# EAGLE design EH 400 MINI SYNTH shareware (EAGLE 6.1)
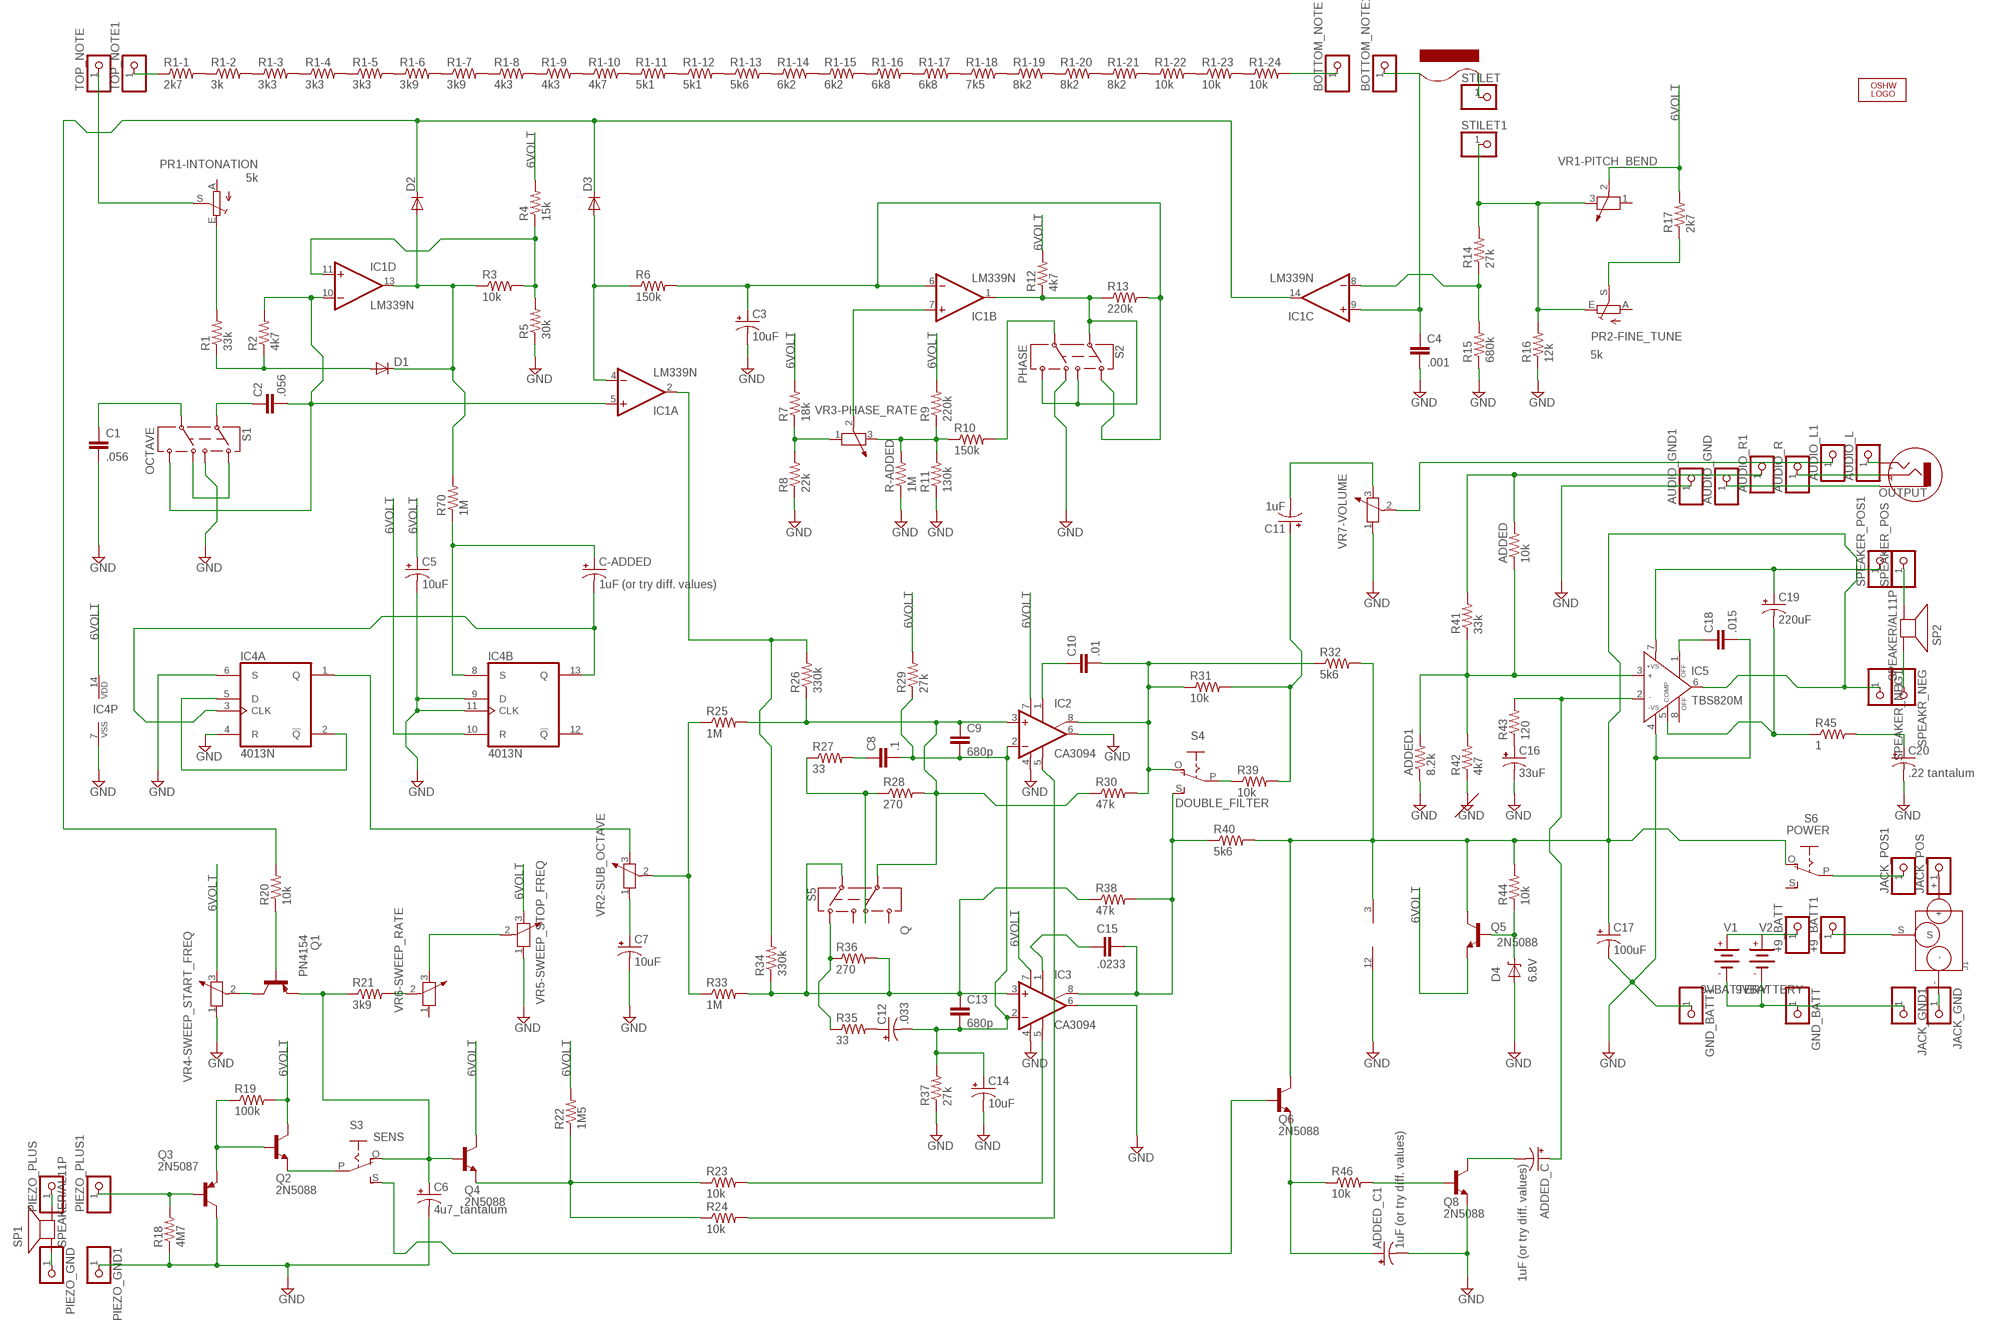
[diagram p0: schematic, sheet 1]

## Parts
+9_BATT  PINHD-1X1  [1X01]
+9_BATT1  PINHD-1X1  [1X01]
ADDED  10k  RESISTORPTH-1/4W  [AXIAL-0.4]
ADDED1  8.2k  RESISTORPTH-1/4W  [AXIAL-0.4]
ADDED_C  1uF (or try diff. values)  CAP_POLPTH2  [CPOL-RADIAL-10UF-25V]
ADDED_C1  1uF (or try diff. values)  CAP_POLPTH2  [CPOL-RADIAL-10UF-25V]
AUDIO_GND  PINHD-1X1  [1X01]
AUDIO_GND1  PINHD-1X1  [1X01]
AUDIO_L  PINHD-1X1  [1X01]
AUDIO_L1  PINHD-1X1  [1X01]
AUDIO_R  PINHD-1X1  [1X01]
AUDIO_R1  PINHD-1X1  [1X01]
BOTTOM_NOTE  PINHD-1X1  [1X01]
BOTTOM_NOTE1  PINHD-1X1  [1X01]
C1  .056  CAP_  [AXIAL-5MM]
C2  .056  CAP_  [AXIAL-5MM]
C3  10uF  CAP_POLPTH1  [CPOL-RADIAL-100UF-25V]
C4  .001  CAP_  [AXIAL-5MM]
C5  10uF  CAP_POLPTH2  [CPOL-RADIAL-10UF-25V]
C6  4u7_tantalum  CAP_POLPTH2  [CPOL-RADIAL-10UF-25V]
C7  10uF  CAP_POLPTH2  [CPOL-RADIAL-10UF-25V]
C8  .1  CAP_  [AXIAL-5MM]
C9  680p  CAP_  [AXIAL-5MM]
C10  .01  CAP_  [AXIAL-5MM]
C11  1uF  CAP_POLPTH1  [CPOL-RADIAL-100UF-25V]
C12  .033  CAP_POLPTH2  [CPOL-RADIAL-10UF-25V]
C13  680p  CAP_  [AXIAL-5MM]
C14  10uF  CAP_POLPTH2  [CPOL-RADIAL-10UF-25V]
C15  .0233  CAPPTH1  [CAP-PTH-5MM]
C16  33uF  CAP_POLPTH2  [CPOL-RADIAL-10UF-25V]
C17  100uF  CAP_POLPTH1  [CPOL-RADIAL-100UF-25V]
C18  .015  CAP_  [AXIAL-5MM]
C19  220uF  CAP_POLPTH1  [CPOL-RADIAL-100UF-25V]
C20  .22 tantalum  CAP_POLPTH1  [CPOL-RADIAL-100UF-25V]
C-ADDED  1uF (or try diff. values)  CAP_POLPTH2  [CPOL-RADIAL-10UF-25V]
D1  DIODE1N4148  [DIODE-1N4148]
D2  DIODE1N4148  [DIODE-1N4148]
D3  DIODE1N4148  [DIODE-1N4148]
D4  6.8V  DIODE-ZENERPTH  [DIODE-ZENER]
GND_BATT  PINHD-1X1  [1X01]
GND_BATT1  PINHD-1X1  [1X01]
IC1  LM339N  [DIL14]
IC2  CA3094  LM3080N  [DIL08]
IC3  CA3094  LM3080N  [DIL08]
IC4  4013N  [DIL14]
IC5  TBS820M  AD744N  [DIL08]
J1  JACK-3.5-3P  [PW-3P-3.5-14X9.5-DIP]
JACK_GND  PINHD-1X1  [1X01]
JACK_GND1  PINHD-1X1  [1X01]
JACK_POS  PINHD-1X1  [1X01]
JACK_POS1  PINHD-1X1  [1X01]
LOGO1  LOGO-OSHW-FILLX0200-NT  [OSHW_FILLX200_NOTEXT]
OUTPUT  AUDIO-JACK2.5MM  [STEREOJACK2.5MM_STEREOJACK2.5MM]
PIEZO_GND  PINHD-1X1  [1X01]
PIEZO_GND1  PINHD-1X1  [1X01]
PIEZO_PLUS  PINHD-1X1  [1X01]
PIEZO_PLUS1  PINHD-1X1  [1X01]
PR1-INTONATION  5k  TRIM_EU-S75P  [S75P]
PR2-FINE_TUNE  5k  TRIM_EU-S75P  [S75P]
Q1  PN4154  2N2907  [TO92-EBC-OVAL]
Q2  2N5088  2N2222  [TO92-EBC-OVAL]
Q3  2N5087  2N2907  [TO92-EBC-OVAL]
Q4  2N5088  2N2222  [TO92-EBC-OVAL]
Q5  2N5088  2N2222  [TO92-EBC-OVAL]
Q6  2N5088  2N2222  [TO92-EBC-OVAL]
Q8  2N5088  2N2222  [TO92-EBC-OVAL]
R1  33k  RESISTORPTH-1/4W  [AXIAL-0.4]
R1-1  2k7  RESISTORAXIAL-0.3  [AXIAL-0.3]
R1-2  3k  RESISTORAXIAL-0.3  [AXIAL-0.3]
R1-3  3k3  RESISTORAXIAL-0.3  [AXIAL-0.3]
R1-4  3k3  RESISTORAXIAL-0.3  [AXIAL-0.3]
R1-5  3k3  RESISTORAXIAL-0.3  [AXIAL-0.3]
R1-6  3k9  RESISTORAXIAL-0.3  [AXIAL-0.3]
R1-7  3k9  RESISTORAXIAL-0.3  [AXIAL-0.3]
R1-8  4k3  RESISTORAXIAL-0.3  [AXIAL-0.3]
R1-9  4k3  RESISTORAXIAL-0.3  [AXIAL-0.3]
R1-10  4k7  RESISTORAXIAL-0.3  [AXIAL-0.3]
R1-11  5k1  RESISTORAXIAL-0.3  [AXIAL-0.3]
R1-12  5k1  RESISTORAXIAL-0.3  [AXIAL-0.3]
R1-13  5k6  RESISTORAXIAL-0.3  [AXIAL-0.3]
R1-14  6k2  RESISTORAXIAL-0.3  [AXIAL-0.3]
R1-15  6k2  RESISTORAXIAL-0.3  [AXIAL-0.3]
R1-16  6k8  RESISTORAXIAL-0.3  [AXIAL-0.3]
R1-17  6k8  RESISTORAXIAL-0.3  [AXIAL-0.3]
R1-18  7k5  RESISTORAXIAL-0.3  [AXIAL-0.3]
R1-19  8k2  RESISTORAXIAL-0.3  [AXIAL-0.3]
R1-20  8k2  RESISTORAXIAL-0.3  [AXIAL-0.3]
R1-21  8k2  RESISTORAXIAL-0.3  [AXIAL-0.3]
R1-22  10k  RESISTORAXIAL-0.3  [AXIAL-0.3]
R1-23  10k  RESISTORAXIAL-0.3  [AXIAL-0.3]
R1-24  10k  RESISTORAXIAL-0.3  [AXIAL-0.3]
R2  4k7  RESISTORPTH-1/4W  [AXIAL-0.4]
R3  10k  RESISTORPTH-1/4W  [AXIAL-0.4]
R4  15k  RESISTORPTH-1/4W  [AXIAL-0.4]
R5  30k  RESISTORPTH-1/4W  [AXIAL-0.4]
R6  150k  RESISTORPTH-1/4W  [AXIAL-0.4]
R7  18k  RESISTORPTH-1/4W  [AXIAL-0.4]
R8  22k  RESISTORPTH-1/4W  [AXIAL-0.4]
R9  220k  RESISTORPTH-1/4W  [AXIAL-0.4]
R10  150k  RESISTORPTH-1/4W  [AXIAL-0.4]
R11  130k  RESISTORPTH-1/4W  [AXIAL-0.4]
R12  4k7  RESISTORPTH-1/4W  [AXIAL-0.4]
R13  220k  RESISTORPTH-1/4W  [AXIAL-0.4]
R14  27k  RESISTORPTH-1/4W  [AXIAL-0.4]
R15  680k  RESISTORPTH-1/4W  [AXIAL-0.4]
R16  12k  RESISTORPTH-1/4W  [AXIAL-0.4]
R17  2k7  RESISTORPTH-1/4W  [AXIAL-0.4]
R18  4M7  RESISTORPTH-1/4W  [AXIAL-0.4]
R19  100k  RESISTORPTH-1/4W  [AXIAL-0.4]
R20  10k  RESISTORPTH-1/4W  [AXIAL-0.4]
R21  3k9  RESISTORPTH-1/4W  [AXIAL-0.4]
R22  1M5  RESISTORPTH-1/4W  [AXIAL-0.4]
R23  10k  RESISTORPTH-1/4W  [AXIAL-0.4]
R24  10k  RESISTORPTH-1/4W  [AXIAL-0.4]
R25  1M  RESISTORPTH-1/4W  [AXIAL-0.4]
R26  330k  RESISTORPTH-1/4W  [AXIAL-0.4]
R27  33  RESISTORPTH-1/4W  [AXIAL-0.4]
R28  270  RESISTORPTH-1/4W  [AXIAL-0.4]
R29  27k  RESISTORPTH-1/4W  [AXIAL-0.4]
R30  47k  RESISTORPTH-1/4W  [AXIAL-0.4]
R31  10k  RESISTORPTH-1/4W  [AXIAL-0.4]
R32  5k6  RESISTORPTH-1/4W  [AXIAL-0.4]
R33  1M  RESISTORPTH-1/4W  [AXIAL-0.4]
R34  330k  RESISTORPTH-1/4W  [AXIAL-0.4]
R35  33  RESISTORPTH-1/4W  [AXIAL-0.4]
R36  270  RESISTORPTH-1/4W  [AXIAL-0.4]
R37  27k  RESISTORPTH-1/4W  [AXIAL-0.4]
R38  47k  RESISTORPTH-1/4W  [AXIAL-0.4]
R39  10k  RESISTORPTH-1/4W  [AXIAL-0.4]
R40  5k6  RESISTORPTH-1/4W  [AXIAL-0.4]
R41  33k  RESISTORPTH-1/4W  [AXIAL-0.4]
R42  4k7  RESISTORPTH-1/4W  [AXIAL-0.4]
R43  120  RESISTORPTH-1/4W  [AXIAL-0.4]
R44  10k  RESISTORPTH-1/4W  [AXIAL-0.4]
R45  1  RESISTORPTH-1/4W  [AXIAL-0.4]
R46  10k  RESISTORPTH-1/4W  [AXIAL-0.4]
R70  1M  RESISTORPTH-1/4W  [AXIAL-0.4]
R-ADDED  1M  RESISTORPTH-1/4W  [AXIAL-0.4]
S1  OCTAVE  SWITCH-DPDTOS  [OS]
S2  PHASE  SWITCH-DPDTOS  [OS]
S3  SENS  EG1218S  [EG1218]
S4  DOUBLE_FILTER  EG1218S  [EG1218]
S5  Q  SWITCH-DPDTOS  [OS]
S6  POWER  EG1218S  [EG1218]
SP1  SPEAKER/AL11P  [AL11P]
SP2  SPEAKER/AL11P  [AL11P]
SPEAKER_NEG1  PINHD-1X1  [1X01]
SPEAKER_POS  PINHD-1X1  [1X01]
SPEAKER_POS1  PINHD-1X1  [1X01]
SPEAKR_NEG  PINHD-1X1  [1X01]
STILET  PINHD-1X1  [1X01]
STILET1  PINHD-1X1  [1X01]
TOP_NOTE  PINHD-1X1  [1X01]
TOP_NOTE1  PINHD-1X1  [1X01]
V1  9VBATTERY  [AB9V]
V2  9VBATTERY  [AB9V]
VR1-PITCH_BEND  10k  R-POTENTIOMETER-3362U  [3362U]
VR2-SUB_OCTAVE  100k  R-POTENTIOMETER-3362U  [3362U]
VR3-PHASE_RATE  100k  R-POTENTIOMETER-3362U  [3362U]
VR4-SWEEP_START_FREQ  10k  R-POTENTIOMETER-3362U  [3362U]
VR5-SWEEP_STOP_FREQ  100k  R-POTENTIOMETER-3362U  [3362U]
VR6-SWEEP_RATE  100k  R-POTENTIOMETER-3362U  [3362U]
VR7-VOLUME  100k  R-POTENTIOMETER-3362U  [3362U]

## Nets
6VOLT: C5.1(+) IC2.7(V+) IC3.7(V+) IC4.10(B:R) IC4.14(P:VDD) Q2.C Q4.C Q5.E R4.P$2 R7.P$2 R9.P$2 R12.P$2 R17.P$2 R19.P$2 R22.P$2 R29.P$2 VR1-PITCH_BEND.2 VR4-SWEEP_START_FREQ.3 VR5-SWEEP_STOP_FREQ.3
GND: ADDED1.P$1 ADDED_C1.2(-) AUDIO_GND1.1 C1.P$2 C3.2(-) C4.P$2 C5.2(-) C6.2(-) C7.2(-) C14.2(-) C16.2(-) C17.2(-) C18.P$2 C20.2(-) D4.P$2(A) GND_BATT1.1 IC1.12(P:GND) IC2.4(V-) IC2.6(OUT) IC3.4(V-) IC3.6(OUT) IC4.4(A:R) IC4.6(A:S) IC4.7(P:VSS) IC4.9(B:D) IC4.11(B:CLK) IC5.4(-VS) PIEZO_GND1.1 Q3.C Q8.E R5.P$1 R8.P$1 R11.P$1 R15.P$1 R16.P$1 R18.P$1 R37.P$1 R42.P$1 R-ADDED.P$1 S1.3 S2.4 VR4-SWEEP_START_FREQ.1 VR5-SWEEP_STOP_FREQ.1 VR7-VOLUME.1
N$1: IC1.7(B:+IN) VR3-PHASE_RATE.2
N$2: C8.P$2 C9.P$2 C12.2(-) C13.P$2 C14.1(+) IC2.2(-IN) IC3.2(-IN) R29.P$1 R37.P$2
N$3: C7.1(+) VR2-SUB_OCTAVE.1
N$4: R7.P$1 R8.P$2 VR3-PHASE_RATE.1
N$5: C3.1(+) IC1.6(B:-IN) R6.P$2 R13.P$2 S2.1
N$6: D3.A IC1.4(A:-IN) R6.P$1
N$7: R10.P$2 S2.5
N$8: R9.P$1 R10.P$1 R11.P$2 R-ADDED.P$2 VR3-PHASE_RATE.3
N$9: IC1.2(A:OUT) R26.P$2 R34.P$2
N$10: D1.A R1.P$1 R2.P$1
N$11: C-ADDED.1(+) IC4.8(B:S) R70.P$1
N$12: AUDIO_L1.1 VR7-VOLUME.2
N$13: PR1-INTONATION.E R1.P$2
N$14: D1.C D2.A IC1.13(D:OUT) R3.P$1 R70.P$2
N$15: D2.C D3.C IC1.14(C:OUT) R20.P$2
N$16: IC1.11(D:+IN) R3.P$2 R4.P$1 R5.P$2
N$17: C-ADDED.2(-) IC4.3(A:CLK) IC4.13(B:Q)
N$18: R1-1.P$1 TOP_NOTE1.1
N$19: R1-1.P$2 R1-2.P$1
N$20: R1-2.P$2 R1-3.P$1
N$21: R1-3.P$2 R1-4.P$1
N$22: R1-4.P$2 R1-5.P$1
N$23: R1-5.P$2 R1-6.P$1
N$24: R1-6.P$2 R1-7.P$1
N$25: R1-7.P$2 R1-8.P$1
N$26: R1-8.P$2 R1-9.P$1
N$27: R1-9.P$2 R1-10.P$1
N$28: R1-10.P$2 R1-11.P$1
N$29: R1-11.P$2 R1-12.P$1
N$30: R1-12.P$2 R1-13.P$1
N$31: R1-15.P$2 R1-16.P$1
N$32: R1-16.P$2 R1-17.P$1
N$33: R1-17.P$2 R1-18.P$1
N$34: R1-18.P$2 R1-19.P$1
N$35: R1-19.P$2 R1-20.P$1
N$36: R1-13.P$2 R1-14.P$1
N$37: R1-14.P$2 R1-15.P$1
N$38: R1-20.P$2 R1-21.P$1
N$39: R1-21.P$2 R1-22.P$1
N$40: R25.P$1 R33.P$1 VR2-SUB_OCTAVE.2
N$41: R35.P$1 R36.P$1 S5.1
N$42: C9.P$1 IC2.3(+IN) R25.P$2 R26.P$1 R28.P$2 R30.P$1 S5.5
N$43: Q1.C VR4-SWEEP_START_FREQ.2
N$44: C13.P$1 IC3.3(+IN) R33.P$2 R34.P$1 R36.P$2 R38.P$1 S5.2
N$45: BOTTOM_NOTE1.1 C4.P$1 IC1.9(C:+IN)
N$46: PR2-FINE_TUNE.S R17.P$1
N$47: IC4.2(A:!Q) IC4.5(A:D)
N$48: IC4.1(A:Q) VR2-SUB_OCTAVE.3
N$49: IC1.1(B:OUT) R12.P$1 R13.P$1 S2.2 S2.3 S2.6
N$50: C1.P$1 S1.5
N$51: C2.P$1 S1.2
N$52: C2.P$2 IC1.5(A:+IN) IC1.10(D:-IN) R2.P$2 S1.6
N$53: S1.1 S1.4
N$54: Q1.B R20.P$1
N$55: C6.1(+) Q1.E Q4.B R21.P$1 S3.O
N$56: R21.P$2 VR6-SWEEP_RATE.2
N$57: VR5-SWEEP_STOP_FREQ.2 VR6-SWEEP_RATE.3
N$58: Q2.E S3.P
N$59: IC2.5(OPT) R24.P$2
N$60: Q2.B Q3.E R19.P$1
N$61: PIEZO_PLUS1.1 Q3.B R18.P$2
N$62: IC3.5(OPT) R23.P$2
N$63: Q4.E R22.P$1 R23.P$1 R24.P$1
N$64: IC1.8(C:-IN) R14.P$1 R15.P$2
N$65: PR2-FINE_TUNE.E R14.P$2 R16.P$2 STILET1.1 VR1-PITCH_BEND.3
N$66: C12.1(+) R35.P$2
N$67: C8.P$1 R27.P$2
N$68: R27.P$1 R28.P$1 S5.4
N$69: C10.P$1 IC2.1(ON1)
N$70: C15.1 IC3.1(ON1)
N$71: C15.2 IC3.8(ON2) R38.P$2 R40.P$1 S4.S
N$72: R39.P$1 S4.P
N$73: C10.P$2 IC2.8(ON2) R30.P$2 R31.P$1 R32.P$1 S4.O
N$74: C11.1(+) R31.P$2 R39.P$2
N$75: C17.1(+) IC1.3(P:V+) IC5.6(OUT) Q5.C Q6.C R32.P$2 R40.P$2 R44.P$2 S6.O SPEAKER_NEG1.1
N$76: C11.2(-) VR7-VOLUME.3
N$77: R1-22.P$2 R1-23.P$1
N$78: ADDED1.P$2 ADDED.P$1 IC5.3(IN+) R41.P$1 R42.P$2
N$79: ADDED.P$2 AUDIO_R1.1 R41.P$2
N$80: C18.P$1 IC5.1(OFF)
N$81: C19.1(+) IC5.7(+VS) SPEAKER_POS1.1
N$82: C19.2(-) IC5.5(COMP) R45.P$1
N$83: STILET.1
N$84: C20.1(+) R45.P$2
N$85: ADDED_C.1(+) IC5.2(IN-) R43.P$2
N$86: C16.1(+) R43.P$1
N$87: PIEZO_GND.1 SP1.+
N$88: PIEZO_PLUS.1 SP1.-
N$89: JACK_POS1.1 S6.P
N$90: +9_BATT.1 V1.+ V2.+
N$91: D4.P$1(C) Q5.B R44.P$1
N$92: SP2.- SPEAKER_POS.1
N$93: SP2.+ SPEAKR_NEG.1
N$94: J1.+ JACK_POS.1
N$95: +9_BATT1.1 J1.S
N$96: GND_BATT.1 JACK_GND1.1 V1.- V2.-
N$97: J1.- JACK_GND.1
N$98: AUDIO_L.1 OUTPUT.SHIELD(LEFT)
N$99: AUDIO_R.1 OUTPUT.TIP(RIGHT)
N$100: AUDIO_GND.1 OUTPUT.RING1(SLEEVE)
N$101: Q6.B S3.S
N$102: ADDED_C1.1(+) Q6.E R46.P$1
N$103: Q8.B R46.P$2
N$104: ADDED_C.2(-) Q8.C
N$105: R1-23.P$2 R1-24.P$1
N$106: BOTTOM_NOTE.1 R1-24.P$2
N$202: PR1-INTONATION.S TOP_NOTE.1
Unconnected: IC4.12(B:!Q) IC5.8(OFF) PR1-INTONATION.A PR2-FINE_TUNE.A S5.3 S5.6 S6.S VR1-PITCH_BEND.1 VR6-SWEEP_RATE.1

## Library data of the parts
+9_BATT +9_BATT1 AUDIO_GND AUDIO_GND1 AUDIO_L AUDIO_L1 AUDIO_R AUDIO_R1 BOTTOM_NOTE BOTTOM_NOTE1 GND_BATT GND_BATT1 JACK_GND JACK_GND1 JACK_POS JACK_POS1 PIEZO_GND PIEZO_GND1 PIEZO_PLUS PIEZO_PLUS1 SPEAKER_NEG1 SPEAKER_POS SPEAKER_POS1 SPEAKR_NEG STILET STILET1 TOP_NOTE TOP_NOTE1 = adafruit:PINHD-1X1: Pin header 1x1 for 0.1" spacing
ADDED ADDED1 R1 R1-1-R1-24 R2-R46 R70 R-ADDED = SparkFun:RESISTOR: Resistor
ADDED_C ADDED_C1 C3 C5-C7 C11 C12 C14 C16 C17 C19 C20 C-ADDED = SparkFun:CAP_POL: Capacitor Polarized
C1 C2 C4 C8-C10 C13 C15 C18 = SparkFun-MIRO:CAP: Capacitor
D1-D3 = SparkFun:DIODE: Diode
D4 = SparkFun:DIODE-ZENER: Zener Diode
IC1 = linear:LM339: Low Power Low Offset Voltage Quad Comparators with open collector; LM139/LM239/LM339/LM2901/LM3302
IC2 IC3 = linear:*3080: OP AMP
IC4 = 40xx:4013: Dual D FLIP FLOP, set/reset
IC5 = analog-devices:AD744: Precision, 500 ns Settling BiFET Op Amp Source: http://www.analog.com/static/imported-files/data_sheets/AD744.pdf; MF: ALTERA CORPORATION; MPN: AD744JNZ; OC_FARNELL: 1438362; OC_NEWARK: 59K4810
J1 = Connector:JACK-3.5-3P
LOGO1 = Logo:LOGO-OSHW-FILL
OUTPUT = SparkFun:AUDIO-JACK: 3.5mm Audio Jack Simple 3.5mm common PCB mount audio jack. SKU: PRT-08032
PR1-INTONATION PR2-FINE_TUNE = pot:TRIM_EU-: POTENTIOMETER
Q1 Q3 = adafruit:2N2907*: PNP Transistor Big Oval pads
Q2 Q4-Q6 Q8 = adafruit:2N2222: NPN TRANSISTOR Big oval pads
S1 S2 S5 = SparkFun-MIRO:SWITCH-DPDT: DPDT Version of the COM-00597
S3 S4 S6 = adafruit:EG1218: SLIDING SWITCH 0.1" spacing through hole, vertical SPDT slide switch http://www.ladyada.net/library/pcb/eaglelibrary.html
SP1 SP2 = adafruit:SPEAKER: SPEAKER
V1 V2 = gm-supply:9VBATTERY
VR1-PITCH_BEND VR2-SUB_OCTAVE VR3-PHASE_RATE VR4-SWEEP_START_FREQ VR5-SWEEP_STOP_FREQ VR6-SWEEP_RATE VR7-VOLUME = Discrete:R-POTENTIOMETER*: Potentiometer

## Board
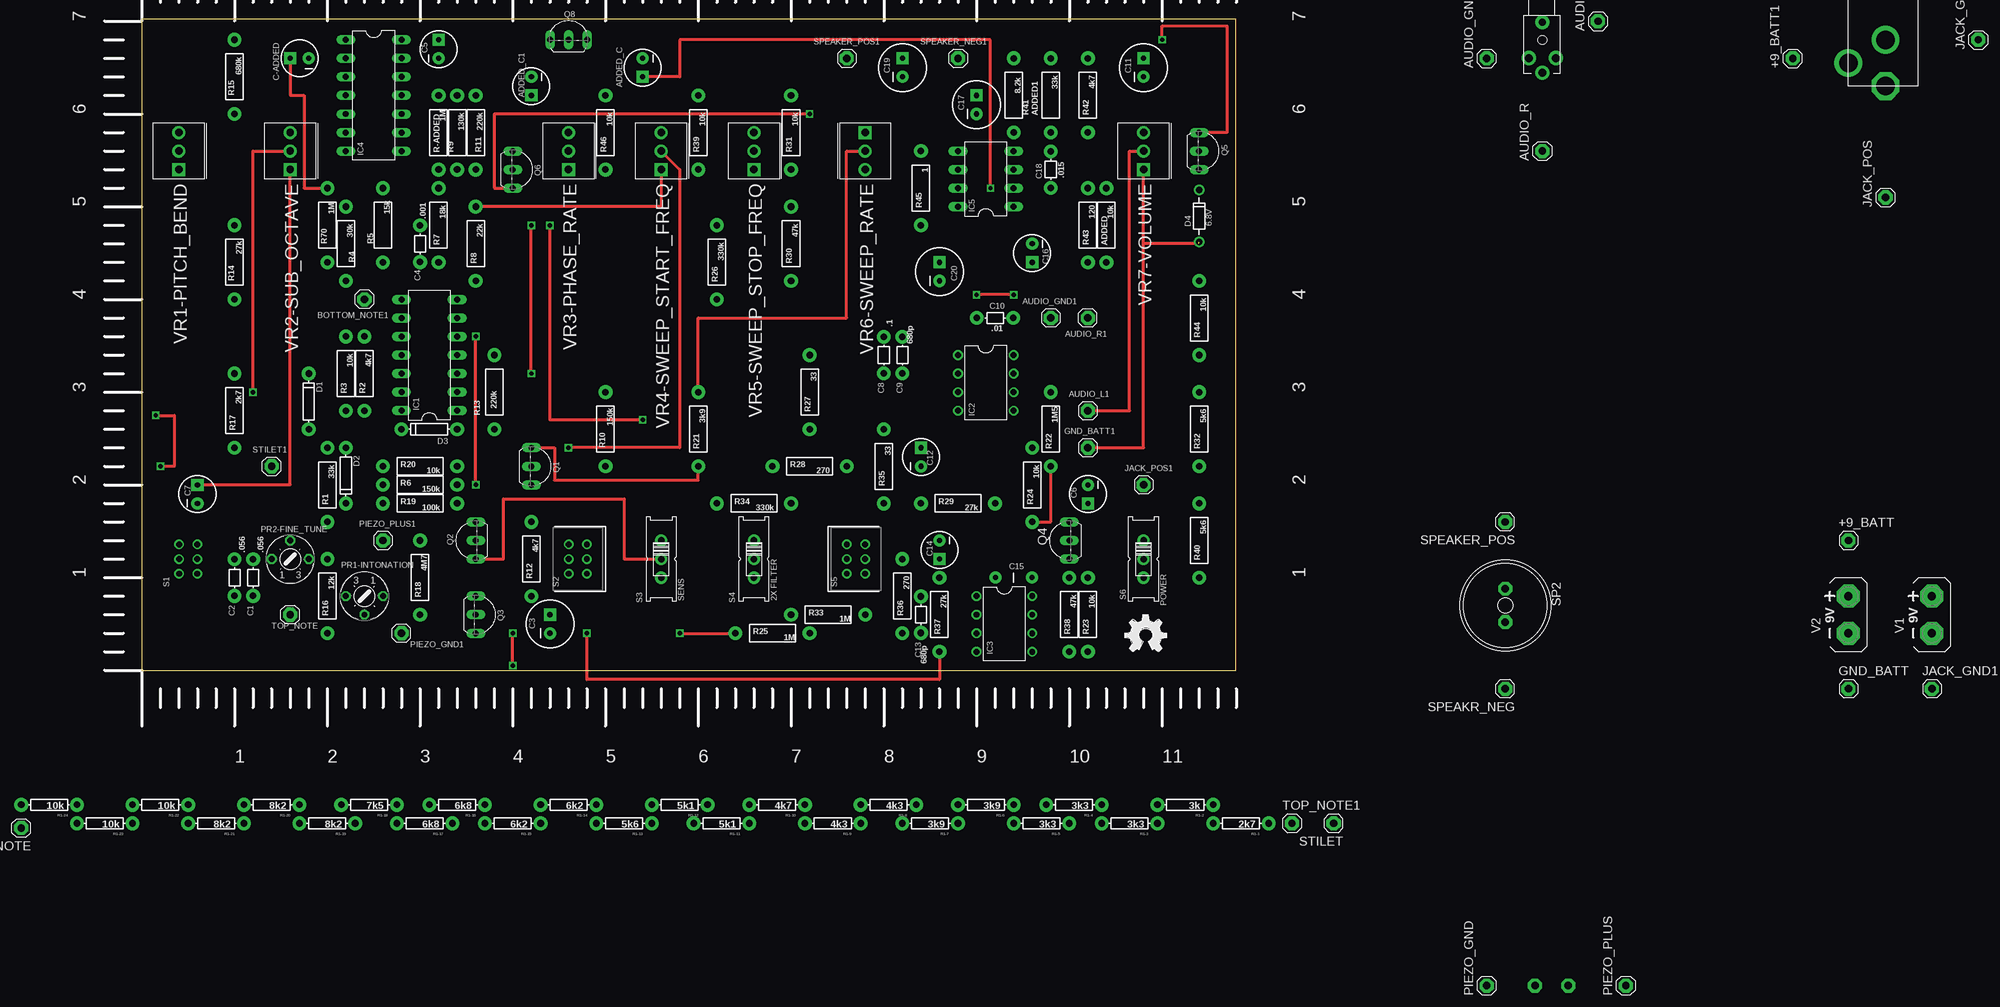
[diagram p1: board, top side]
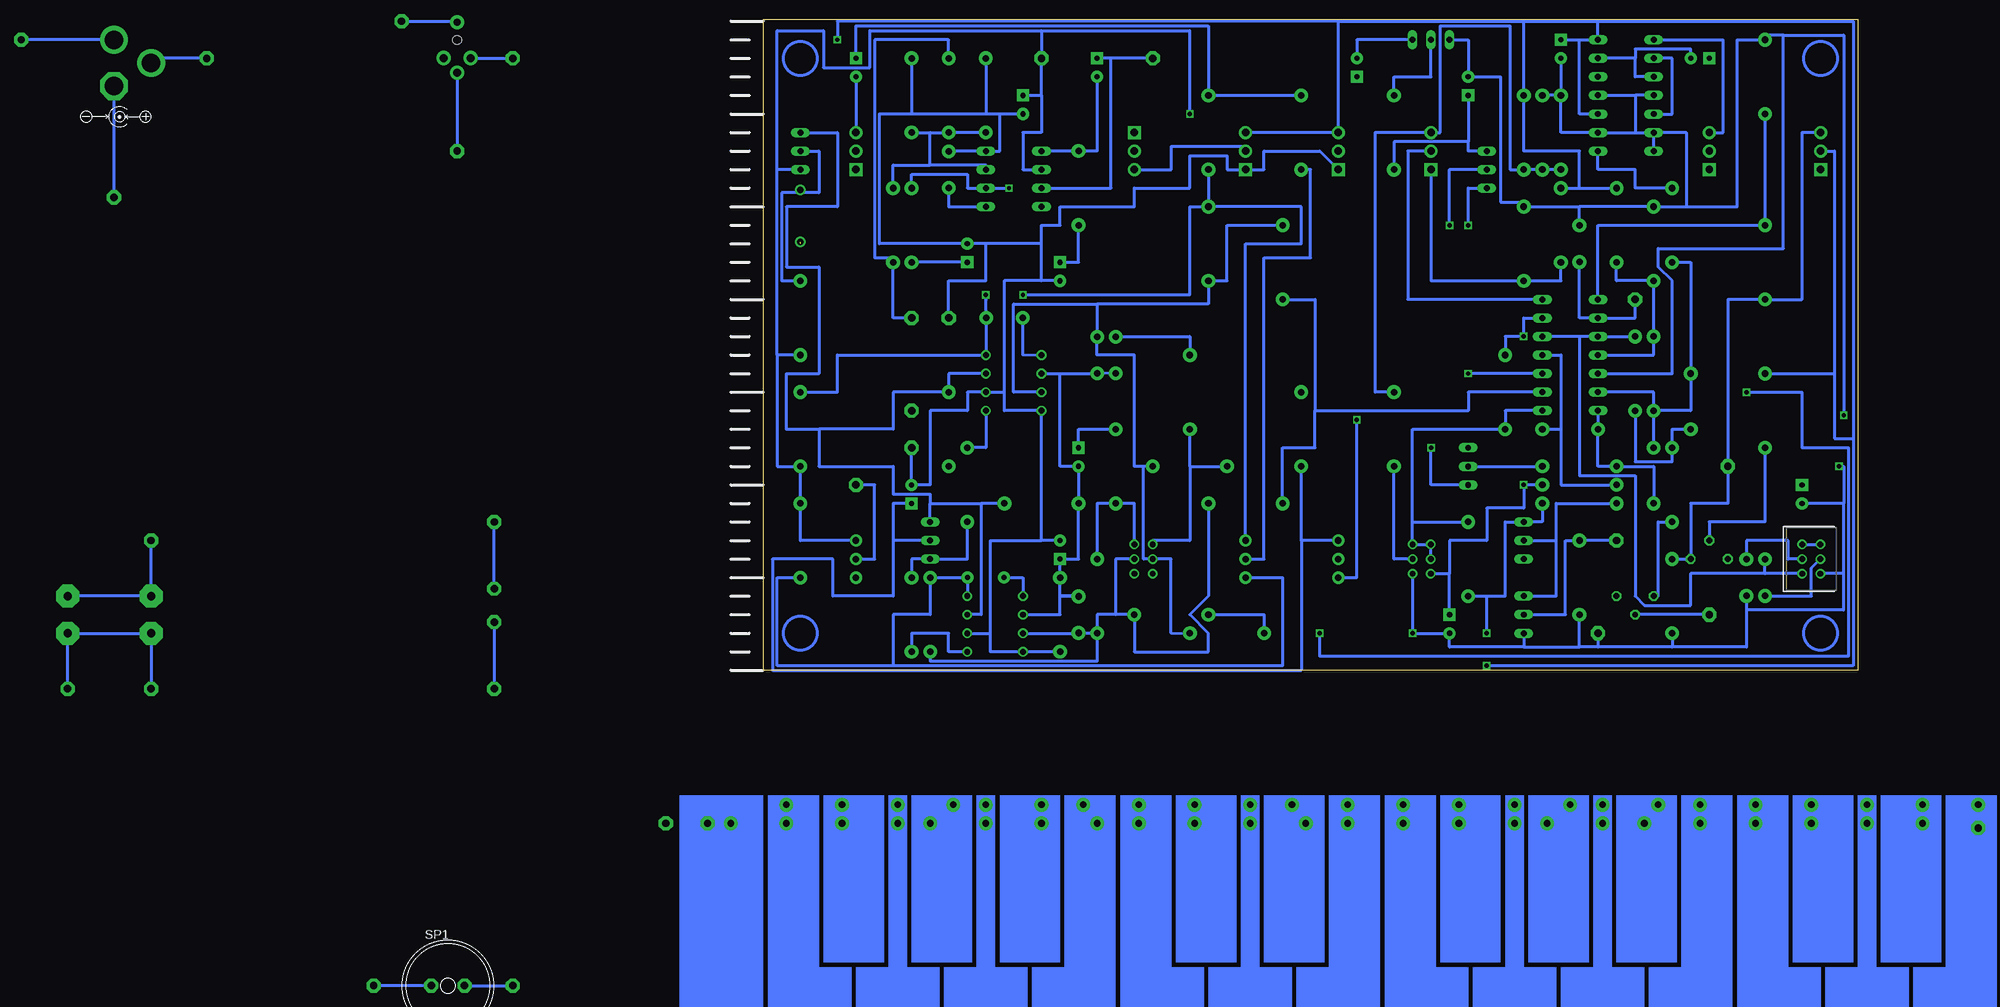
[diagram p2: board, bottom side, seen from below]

Size 149.84 x 89.2 mm. Coordinates in mm from the lower left corner, seen from the top.
Outline: 0,0 149.84,0 149.84,89.2 0,89.2 0,0
Copper layers (1*16): Top 0.035mm / dielectric 1.5mm / Bottom 0.035mm
Design rules: minimum track width 10mil, minimum drill 24mil, track to track 8mil, track to pad 8mil, pad to pad 8mil, via to via 8mil, smd to smd 8mil, copper to edge 40mil, drill to drill 8mil, minimum pad ring 10mil, minimum via ring 8mil, stop-mask expansion 4mil, vias tented up to drill 0mil, thermal gap 10mil

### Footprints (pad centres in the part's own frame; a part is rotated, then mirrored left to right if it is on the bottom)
1X01 = drill 1.016 pad 1.93 octagon: 1 0,0
AXIAL-0.4 = drill 0.9 pad 1.88: P$1 -5.08,0; P$2 5.08,0
CPOL-RADIAL-10UF-25V = drill 0.7 pad 1.651 square: 1 1.27,0 | drill 0.7 pad 1.651: 2 -1.27,0
AXIAL-5MM = drill 0.9 pad 1.88: P$1 -2.5,0; P$2 2.5,0
CPOL-RADIAL-100UF-25V = drill 0.7 pad 1.651 square: 1 1.27,0 | drill 0.7 pad 1.651: 2 -1.27,0
CAP-PTH-5MM = drill 0.7 pad 1.651: 1 -2.5,0; 2 2.5,0
DIODE-1N4148 = drill 0.9 pad 1.88: A -3.81,0; C 3.81,0
DIODE-ZENER = drill 0.9: P$1 -3.556,0; P$2 3.556,0
DIL14 = drill 0.813 long: 1 -7.62,-3.81; 2 -5.08,-3.81; 3 -2.54,-3.81; 4 0,-3.81; 5 2.54,-3.81; 6 5.08,-3.81; 7 7.62,-3.81; 8 7.62,3.81; 9 5.08,3.81; 10 2.54,3.81; 11 0,3.81; 12 -2.54,3.81; 13 -5.08,3.81; 14 -7.62,3.81
DIL08 = drill 0.813 pad 1.27: 1 -3.81,-3.81; 2 -1.27,-3.81; 3 1.27,-3.81; 4 3.81,-3.81; 5 3.81,3.81; 6 1.27,3.81; 7 -1.27,3.81; 8 -3.81,3.81
DIL08' = drill 0.813 long: 1 -3.81,-3.81; 2 -1.27,-3.81; 3 1.27,-3.81; 4 3.81,-3.81; 5 3.81,3.81; 6 1.27,3.81; 7 -1.27,3.81; 8 -3.81,3.81
PW-3P-3.5-14X9.5-DIP = drill 2.54 pad 3.81 octagon: + 0,0 | drill 2.54 pad 3.81: - -6.35,0; S -3.175,-5.08
STEREOJACK2.5MM_STEREOJACK2.5MM = drill 1.1 pad 1.93: RING1 2.5,-1.85; RING2 2.5,1.85; TIP 4.5,0 | drill 1 pad 1.93: SHIELD -2.4,0 | hole 1.2: 0,0
S75P = drill 0.813 octagon: A -2.54,0; E 2.54,0; S 0,2.54
TO92-EBC-OVAL = drill 0.813 long: B 0,-1.27; C 2.54,-1.27; E -2.54,-1.27
AXIAL-0.3 = drill 0.9 pad 1.88: P$1 -3.81,0; P$2 3.81,0
OS = drill 0.787 pad 1.27: 1 -2.007,1.245; 2 0,1.245; 3 2.007,1.245; 4 -2.007,-1.245; 5 0,-1.245; 6 2.007,-1.245
EG1218 = drill 0.9 pad 1.676: O -2.54,0; P 0,0; S 2.54,0
AL11P = drill 1.016 pad 1.905 octagon: + 2.286,0; - -2.286,0
AB9V = drill 1.118 pad 3.15 octagon: + 0,2.54; - 0,-2.54
3362U = drill 1.016 pad 1.778 square: 1 0,2.54 | drill 1.016 pad 1.778: 2 2.54,2.54; 3 5.08,2.54

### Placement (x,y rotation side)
+9_BATT  233.68,17.78 0 top  (outside the outline)
+9_BATT1  226.06,83.82 90 top  (outside the outline)
ADDED  132.08,60.96 270 top
ADDED1  119.38,78.74 270 top
ADDED_C  68.58,82.55 270 top
ADDED_C1  53.34,80.01 270 top
AUDIO_GND  184.15,83.82 90 top  (outside the outline)
AUDIO_GND1  124.46,48.26 0 top
AUDIO_L  199.39,88.9 90 top  (outside the outline)
AUDIO_L1  129.54,35.56 0 top
AUDIO_R  191.77,71.12 90 top  (outside the outline)
AUDIO_R1  129.54,48.26 180 top
BOTTOM_NOTE  -16.51,-21.59 180 top  (outside the outline)
BOTTOM_NOTE1  30.48,50.8 270 top
C1  15.24,12.7 270 top
C2  12.7,12.7 90 top
C3  55.88,6.35 90 top
C4  38.1,58.42 90 top
C5  40.64,85.09 90 top
C6  129.54,24.13 270 top
C7  7.62,24.13 90 top
C8  101.6,43.18 270 top
C9  104.14,43.18 270 top
C10  116.84,48.26 0 top
C11  137.16,82.55 90 top
C12  106.68,29.21 90 top
C13  106.68,7.62 90 top
C14  109.22,16.51 270 top
C15  119.38,12.7 0 top
C16  121.92,57.15 270 top
C17  114.3,77.47 90 top
C18  124.46,68.58 90 top
C19  104.14,82.55 90 top
C20  109.22,54.61 90 top
C-ADDED  21.59,83.82 180 top
D1  22.86,36.83 90 top
D2  27.94,26.67 270 top
D3  39.37,33.02 180 top
D4  144.78,62.23 270 top
GND_BATT  233.68,-2.54 0 top  (outside the outline)
GND_BATT1  129.54,30.48 0 top
IC1  39.37,43.18 90 top
IC2  115.57,39.37 270 top
IC3  118.11,6.35 270 top
IC4  31.75,78.74 270 top
IC5  TBS820M  [DIL08']  115.57,67.31 90 top
J1  238.76,80.01 270 top  (outside the outline)
JACK_GND  251.46,86.36 90 top  (outside the outline)
JACK_GND1  245.11,-2.54 0 top  (outside the outline)
JACK_POS  238.76,64.77 90 top  (outside the outline)
JACK_POS1  137.16,25.4 0 top
LOGO1  134.62,2.54 0 top
OUTPUT  191.77,86.36 270 top  (outside the outline)
PIEZO_GND  184.15,-43.18 90 top  (outside the outline)
PIEZO_GND1  35.56,5.08 180 top
PIEZO_PLUS  203.2,-43.18 90 top  (outside the outline)
PIEZO_PLUS1  33.02,17.78 0 top
PR1-INTONATION  30.48,10.16 180 top
PR2-FINE_TUNE  20.32,15.24 0 top
Q1  54.61,27.94 270 top
Q2  44.45,17.78 90 top
Q3  46.99,7.62 270 top
Q4  125.73,17.78 90 top
Q5  146.05,71.12 270 top
Q6  52.07,68.58 270 top
Q8  58.42,87.63 0 top
R1  25.4,25.4 270 top
R1-1  150.5,-20.96 180 top  (outside the outline)
R1-2  142.88,-18.41 180 top  (outside the outline)
R1-3  135.25,-20.96 180 top  (outside the outline)
R1-4  127.64,-18.41 180 top  (outside the outline)
R1-5  123.19,-20.96 180 top  (outside the outline)
R1-6  115.57,-18.41 180 top  (outside the outline)
R1-7  107.95,-20.96 180 top  (outside the outline)
R1-8  102.23,-18.41 180 top  (outside the outline)
R1-9  94.61,-20.96 180 top  (outside the outline)
R1-10  87,-18.41 180 top  (outside the outline)
R1-11  79.38,-20.96 180 top  (outside the outline)
R1-12  73.66,-18.41 180 top  (outside the outline)
R1-13  66.04,-20.96 180 top  (outside the outline)
R1-14  58.42,-18.41 180 top  (outside the outline)
R1-15  50.8,-20.96 180 top  (outside the outline)
R1-16  43.18,-18.41 180 top  (outside the outline)
R1-17  38.73,-20.96 180 top  (outside the outline)
R1-18  31.11,-18.41 180 top  (outside the outline)
R1-19  25.4,-20.96 180 top  (outside the outline)
R1-20  17.78,-18.41 180 top  (outside the outline)
R1-21  10.16,-20.96 180 top  (outside the outline)
R1-22  2.54,-18.41 180 top  (outside the outline)
R1-23  -5.08,-20.96 180 top  (outside the outline)
R1-24  -12.7,-18.41 180 top  (outside the outline)
R2  30.48,40.64 90 top
R3  27.94,40.64 90 top
R4  33.02,60.96 90 top
R5  27.94,58.42 270 top
R6  38.1,25.4 0 top
R7  40.64,60.96 90 top
R8  45.72,58.42 270 top
R9  45.72,73.66 90 top
R10  63.5,33.02 270 top
R11  43.18,73.66 270 top
R12  53.34,15.24 270 top
R13  48.26,38.1 90 top
R14  12.7,55.88 270 top
R15  12.7,81.28 270 top
R16  25.4,10.16 90 top
R17  12.7,35.56 90 top
R18  38.1,12.7 90 top
R19  38.1,22.86 0 top
R20  38.1,27.94 180 top
R21  76.2,33.02 90 top
R22  124.46,33.02 90 top
R23  129.54,7.62 270 top
R24  121.92,25.4 90 top
R25  86.36,5.08 0 top
R26  78.74,55.88 270 top
R27  91.44,38.1 90 top
R28  91.44,27.94 0 top
R29  111.76,22.86 0 top
R30  88.9,58.42 90 top
R31  88.9,73.66 90 top
R32  144.78,33.02 270 top
R33  93.98,7.62 0 top
R34  83.82,22.86 180 top
R35  101.6,27.94 90 top
R36  104.14,10.16 270 top
R37  109.22,7.62 90 top
R38  127,7.62 90 top
R39  76.2,73.66 90 top
R40  144.78,17.78 90 top
R41  124.46,78.74 90 top
R42  129.54,78.74 270 top
R43  129.54,60.96 90 top
R44  144.78,48.26 270 top
R45  106.68,66.04 270 top
R46  63.5,73.66 90 top
R70  25.4,60.96 270 top
R-ADDED  40.64,73.66 270 top
S1  6.35,15.24 270 bottom
S2  59.69,15.24 90 top
S3  71.12,15.24 270 top
S4  83.82,15.24 270 top
S5  97.79,15.24 270 top
S6  137.16,15.24 270 top
SP1  193.04,-43.18 0 bottom  (outside the outline)
SP2  186.69,8.89 270 top  (outside the outline)
SPEAKER_NEG1  111.76,83.82 0 top
SPEAKER_POS  186.69,20.32 180 top  (outside the outline)
SPEAKER_POS1  96.52,83.82 0 top
SPEAKR_NEG  186.69,-2.54 180 top  (outside the outline)
STILET  not placed on the board
STILET1  17.78,27.94 90 top
TOP_NOTE  20.32,7.62 180 top
TOP_NOTE1  157.48,-20.96 0 top  (outside the outline)
V1  245.11,7.62 0 top  (outside the outline)
V2  233.68,7.62 0 top  (outside the outline)
VR1-PITCH_BEND  7.62,68.58 90 top
VR2-SUB_OCTAVE  22.86,68.58 90 top
VR3-PHASE_RATE  60.96,68.58 90 top
VR4-SWEEP_START_FREQ  73.66,68.58 90 top
VR5-SWEEP_STOP_FREQ  86.36,68.58 90 top
VR6-SWEEP_RATE  96.52,73.66 270 top
VR7-VOLUME  139.7,68.58 90 top

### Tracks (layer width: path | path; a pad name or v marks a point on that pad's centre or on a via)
6VOLT  (via drill 0.6)
  Top 0.406: v139.7,86.36 139.7,88.27 148.59,88.27 148.59,73.66 Q5.E | v50.8,0.64 v50.8,5.08
  Bottom 0.406: Q5.E 139.7,73.66 139.7,63.5 146.69,63.5 146.69,55.25 142.24,55.25 142.24,40.64 146.69,40.64 146.69,33.02 142.24,33.02 | 127,22.86 127,24.13 132.08,24.13 132.08,27.94 142.24,27.94 142.24,33.02 | Q4.C 127,22.86 | 127,22.86 120.02,22.86 | R29.P$2 120.02,22.86 | 120.02,22.86 120.02,7.62 IC3.7 | IC2.7 124.46,40.64 R22.P$2 132.08,38.1 132.08,33.02 142.24,33.02 | 71.12,88.9 VR4-SWEEP_START_FREQ.3 VR5-SWEEP_STOP_FREQ.3 | 71.12,88.9 139.7,88.9 v139.7,86.36 | C5.1 38.1,86.36 | R19.P$2 43.18,20.32 Q2.C 48.26,20.32 48.26,10.16 50.8,10.16 | 45.72,88.9 35.56,88.9 | 35.56,88.9 0.64,88.9 0.64,31.75 | 38.1,66.04 38.1,71.12 45.72,71.12 R9.P$2 45.72,88.9 | VR1-PITCH_BEND.2 3.17,71.12 3.17,40.64 | 3.17,40.64 3.17,31.75 0.64,31.75 | 0.64,31.75 0.64,0.64 v50.8,0.64 | 71.12,88.9 45.72,88.9 | IC4.10 38.1,76.2 38.1,86.36 | 38.1,86.36 IC4.14 35.56,88.9 | R12.P$2 50.8,10.16 | v50.8,5.08 50.8,10.16 | R7.P$2 38.1,66.04 | 38.1,66.04 R4.P$2 | R17.P$2 3.17,40.64
GND  (via drill 0.6)  (1 unrouted)
  Top 0.406: v1.91,34.93 4.45,34.93 4.45,27.94 v2.54,27.94 | R37.P$1 109.22,-1.27 60.96,-1.27 v60.96,5.08 | GND_BATT1.1 137.16,30.48 137.16,58.42 | 137.16,58.42 VR7-VOLUME.1 | VR4-SWEEP_START_FREQ.1 71.12,63.5 R8.P$1 | 144.78,58.42 137.16,58.42
  Bottom 0.406: IC4.7 IC4.6 | IC4.4 30.48,78.74 | 30.48,78.74 30.48,73.66 | 30.48,73.66 IC4.6 | R-ADDED.P$1 40.64,73.66 IC4.9 30.48,73.66 | IC4.11 30.48,78.74 | IC4.6 23.5,73.66 23.5,63.5 | 10.16,86.99 1.91,86.99 v1.91,34.93 | v2.54,27.94 1.91,27.94 1.91,22.86 | IC1.12 25.4,40.64 25.4,53.34 27.3,55.25 27.3,57.79 10.16,57.79 10.16,86.99 | 10.16,86.99 12.7,86.99 R15.P$1 16.51,86.36 16.51,63.5 23.5,63.5 | 38.1,63.5 R8.P$1 45.72,64.13 48.9,64.13 48.9,81.28 ADDED_C1.2 53.34,86.36 Q8.E | 23.5,63.5 R5.P$1 38.1,63.5 | C5.2 R-ADDED.P$1 | R-ADDED.P$1 R11.P$1 | C4.P$2 38.1,63.5 | 1.91,22.86 C7.2 8.26,22.86 | 1.91,13.33 1.91,22.86 | 15.24,8.25 1.91,8.25 1.91,13.33 | C1.P$2 15.24,8.25 | 15.24,8.25 15.24,3.17 25.4,3.17 | R16.P$1 25.4,3.17 | 25.4,3.17 35.56,3.17 | PIEZO_GND1.1 35.56,3.17 | 45.72,3.17 38.1,3.17 | 35.56,3.17 38.1,3.17 | 38.1,3.17 R18.P$1 | Q3.C 45.72,3.17 | 45.72,3.17 55.88,3.17 C3.2 v60.96,5.08 | 60.96,4.95 v60.96,5.08 | v60.96,5.08 60.94,5.1 S2.4 | 117.47,76.2 117.47,71.12 IC5.4 124.46,71.12 C18.P$2 | C17.2 117.47,76.2 | 117.47,76.2 119.38,76.2 | 119.38,76.2 129.54,76.2 | R42.P$1 129.54,76.2 | 129.54,76.2 133.99,76.2 133.99,58.42 C16.2 119.38,58.42 | 111.76,53.34 116.84,53.34 116.84,38.1 | 111.76,53.34 111.76,58.42 | 111.76,58.42 119.38,58.42 | C20.2 111.76,53.34 | 111.76,58.42 111.76,60.96 109.22,60.96 109.22,63.5 99.06,63.5 99.06,66.04 91.44,66.04 91.44,70.48 86.36,70.48 86.36,68.58 VR5-SWEEP_STOP_FREQ.1 81.28,68.58 81.28,71.12 73.66,71.12 VR4-SWEEP_START_FREQ.1 | IC3.6 118.75,5.08 | 118.75,5.08 118.75,2.54 IC3.4 R37.P$1 | 118.75,5.08 118.75,17.78 111.76,17.78 | C14.2 111.76,17.78 | 111.76,17.78 IC2.4 116.84,35.56 116.84,38.1
  Bottom 0.406: 116.84,38.1 IC2.6 121.92,38.1 121.92,35.56 127,35.56 127,25.4 C6.2 GND_BATT1.1 | ADDED1.P$1 119.38,76.2 | AUDIO_GND1.1 124.46,53.34 119.38,53.34 119.38,58.42 | S1.3 5.11,13.33 1.91,13.33
N$1
  Bottom 0.406: IC1.7 61.59,50.8 61.59,71.12 VR3-PHASE_RATE.2
N$2
  Bottom 0.406: 109.22,10.16 C13.P$2 106.68,10.16 109.22,10.16 | IC3.2 109.22,7.62 109.22,10.16 | 109.22,10.16 R37.P$2 C14.1 106.68,15.24 R29.P$1 C12.2 109.22,27.94 109.22,40.64 | 109.22,40.64 C9.P$2 | C8.P$2 101.6,40.64 C9.P$2 | IC2.2 109.22,40.64 | 109.22,40.64 104.14,40.64 C9.P$2
N$3
  Top 0.406: VR2-SUB_OCTAVE.1 20.32,25.4 C7.1
N$4
  Bottom 0.406: VR3-PHASE_RATE.1 58.42,53.34 R8.P$2 40.64,53.34 R7.P$1
N$5  (via drill 0.6)
  Top 0.406: v45.72,25.4 v45.72,45.72
  Bottom 0.406: IC1.6 45.72,48.26 v45.72,45.72 48.26,45.72 R13.P$2 | R6.P$2 v45.72,25.4 45.72,22.22 50.8,22.22 50.8,17.78 55.88,17.78 55.88,13.23 | S2.1 55.88,13.23 | C3.1 55.88,13.23
N$6
  Bottom 0.406: IC1.4 40.64,43.18 40.64,33.02 | D3.A 40.64,33.02 | 40.64,33.02 40.64,25.4 R6.P$1
N$7
  Bottom 0.406: S2.5 63.5,15.24 R10.P$2
N$8
  Bottom 0.406: R-ADDED.P$2 R11.P$2 R9.P$1 47.62,68.58 47.62,88.27 57.15,88.27 57.15,73.66 VR3-PHASE_RATE.3 66.04,73.66 66.04,38.1 R10.P$1
N$9
  Bottom 0.406: IC1.2 53.34,38.1 53.34,35.56 74.3,35.56 | R26.P$2 74.3,50.8 74.3,35.56 | R34.P$2 78.74,30.48 74.3,30.48 74.3,35.56
N$10
  Bottom 0.406: D1.A 25.4,33.02 R1.P$1 25.4,28.57 30.48,28.57 R2.P$1
N$11
  Top 0.406: C-ADDED.1 20.32,78.74 22.23,78.74 22.23,66.04 R70.P$1
  Bottom 0.406: R70.P$1 30.48,66.04 30.48,68.58 35.56,68.58 IC4.8
N$12
  Top 0.406: AUDIO_L1.1 135.25,35.56 135.25,71.12 VR7-VOLUME.2
N$13
  Bottom 0.406: PR1-INTONATION.E 27.3,10.16 27.3,20.32 R1.P$2
N$14
  Bottom 0.406: R3.P$1 27.94,38.1 IC1.13 | R70.P$2 22.86,55.88 D1.C 22.86,35.56 R3.P$1 | D2.A R3.P$1
N$15
  Bottom 0.406: D2.C 27.94,27.94 R20.P$2 35.56,27.94 D3.C IC1.14
N$16
  Bottom 0.406: IC1.11 27.94,43.18 R3.P$2 R5.P$2 33.02,53.34 R4.P$1
N$17
  Bottom 0.406: IC4.3 30.48,81.28 30.48,83.82 | 30.48,83.82 IC4.13 | C-ADDED.2 22.86,85.09 30.48,85.09 30.48,83.82
N$18
  Bottom 0.406: TOP_NOTE1.1 R1-1.P$1
N$19
  Bottom 0.406: R1-1.P$2 R1-2.P$1
N$20
  Bottom 0.406: R1-2.P$2 R1-3.P$1
N$21
  Bottom 0.406: R1-3.P$2 R1-4.P$1
N$22
  Bottom 0.406: R1-4.P$2 127,-18.41 R1-5.P$1
N$23
  Bottom 0.406: R1-6.P$1 R1-5.P$2
N$24
  Bottom 0.406: R1-7.P$1 R1-6.P$2
N$25
  Bottom 0.406: R1-8.P$1 104.14,-18.41 R1-7.P$2
N$26
  Bottom 0.406: R1-8.P$2 R1-9.P$1
N$27
  Bottom 0.406: R1-9.P$2 R1-10.P$1
N$28
  Bottom 0.406: R1-10.P$2 R1-11.P$1
N$29
  Bottom 0.406: R1-12.P$1 75.56,-18.41 R1-11.P$2
N$30
  Bottom 0.406: R1-12.P$2 R1-13.P$1
N$31
  Bottom 0.406: R1-16.P$1 R1-15.P$2
N$32
  Bottom 0.406: R1-16.P$2 42.55,-18.41 R1-17.P$1
N$33
  Bottom 0.406: R1-17.P$2 R1-18.P$1
N$34
  Bottom 0.406: R1-18.P$2 29.21,-18.41 R1-19.P$1
N$35
  Bottom 0.406: R1-20.P$1 R1-19.P$2
N$36
  Bottom 0.406: R1-14.P$1 R1-13.P$2
N$37
  Bottom 0.406: R1-14.P$2 R1-15.P$1
N$38
  Bottom 0.406: R1-20.P$2 R1-21.P$1
N$39
  Bottom 0.406: R1-22.P$1 R1-21.P$2
N$40  (via drill 0.6)
  Top 0.406: v73.66,5.08 R25.P$1 | v15.24,38.1 15.24,71.12 VR2-SUB_OCTAVE.2
  Bottom 0.406: v15.24,38.1 7.62,38.1 7.62,30.48 1.27,30.48 1.27,1.91 73.66,1.91 v73.66,5.08 | R33.P$1 81.28,7.62 R25.P$1
N$41
  Bottom 0.406: R36.P$1 104.14,22.86 R35.P$1 99.03,22.86 S5.1
N$42
  Bottom 0.406: IC2.3 115.57,38.1 115.57,50.16 104.14,50.16 | 104.14,50.16 C9.P$1 104.18,43.18 99.06,43.18 99.06,27.94 97.79,27.94 | 104.14,50.16 88.9,50.16 R30.P$1 86.36,53.34 86.36,60.96 R26.P$1 | R28.P$2 97.79,27.94 | 97.79,27.94 97.79,15.24 S5.5 93.98,15.24 94,15.21 94,5.1 R25.P$2
N$43  (via drill 0.6)
  Top 0.406: VR4-SWEEP_START_FREQ.2 73.66,68.58 73.66,30.48 v58.42,30.48
  Bottom 0.406: Q1.C 58.42,25.4 v58.42,30.48
N$44
  Bottom 0.406: R38.P$1 127,1.27 104.14,1.27 R36.P$2 | IC3.3 107.28,5.08 | R36.P$2 106.68,5.08 | 106.68,5.08 C13.P$1 107.28,5.08 | S5.2 101.6,15.24 101.6,7.62 | 101.6,7.62 104.14,7.62 R36.P$2 | 106.68,5.08 107.28,5.08 | 101.6,7.62 R33.P$2 99.06,2.54 88.9,2.54 88.9,5.08 91.44,7.62 88.9,10.16 R34.P$1
N$45
  Bottom 0.406: C4.P$1 38.1,48.26 IC1.9 30.48,48.26 BOTTOM_NOTE1.1
N$46
  Bottom 0.406: R17.P$1 12.7,20.32 20.32,20.32 PR2-FINE_TUNE.S
N$47
  Bottom 0.406: IC4.5 25.4,76.2 25.4,83.82 IC4.2
N$48
  Bottom 0.406: IC4.1 18.41,86.36 18.41,73.66 VR2-SUB_OCTAVE.3
N$49
  Bottom 0.406: 60.96,20.32 60.96,33.02 R13.P$1 48.26,35.56 IC1.1 | 60.96,20.32 60.96,17.14 58.32,17.25 S2.3 | 60.96,20.32 R12.P$1 | S2.6 S2.3 | S2.2 S2.3
N$50
  Bottom 0.406: S1.5 9.53,15.24 9.53,17.78 15.24,17.78 C1.P$1
N$51
  Bottom 0.406: S1.2 6.35,13.99 6.35,10.16 12.7,10.16 | 12.7,10.16 12.7,9.56 | C2.P$1 12.7,10.16
N$52
  Bottom 0.406: 38.1,45.72 IC1.10 R2.P$2 | 38.1,45.72 IC1.5 | 38.1,45.72 38.1,26.67 30.48,26.67 30.48,10.16 29.21,8.89 22.86,8.89 22.86,13.23 12.7,13.23 | S1.6 12.7,13.23 | 12.7,13.23 C2.P$2
N$53
  Bottom 0.406: S1.4 S1.1
N$54
  Bottom 0.406: Q1.B R20.P$1
N$55
  Top 0.406: Q1.E 56.52,30.48 56.52,26.04 76.2,26.04 R21.P$1
  Bottom 0.406: C6.1 132.08,22.86 132.08,17.78 | Q4.B 132.08,17.78 | 132.08,17.78 132.08,10.16 140.34,10.16 140.34,15.24 148.59,15.24 148.59,0 76.2,0 76.2,17.78 | 76.2,17.78 R21.P$1 | S3.O 76.2,17.78
N$56
  Top 0.406: R21.P$2 76.2,48.26 96.52,48.26 96.52,71.12 VR6-SWEEP_RATE.2
N$57
  Bottom 0.406: VR6-SWEEP_RATE.3 93.98,68.58 93.98,71.75 83.82,71.75 VR5-SWEEP_STOP_FREQ.2
N$58
  Top 0.406: Q2.E 49.53,15.24 49.53,23.49 66.04,23.49 66.04,15.24 S3.P
N$59
  Bottom 0.406: IC2.5 119.38,30.48 R24.P$2
N$60
  Bottom 0.406: Q2.B 41.27,17.78 | 41.27,17.78 41.27,22.86 R19.P$1 | Q3.E 41.27,10.16 41.27,17.78
N$61
  Bottom 0.406: Q3.B 40.01,7.62 40.01,17.78 R18.P$2 PIEZO_PLUS1.1
N$62
  Bottom 0.406: IC3.5 124.46,2.54 124.46,5.08 129.54,5.08 R23.P$2
N$63
  Top 0.406: R24.P$1 124.46,20.32 R22.P$1
  Bottom 0.406: R23.P$1 129.54,15.24 Q4.E 121.92,15.24 R24.P$1
N$64
  Bottom 0.406: IC1.8 35.56,60.96 R14.P$1 R15.P$2
N$65
  Bottom 0.406: VR1-PITCH_BEND.3 7.62,73.66 7.62,50.8 R14.P$2 17.78,50.8 STILET1.1 17.78,22.86 22.86,22.86 PR2-FINE_TUNE.E R16.P$2
N$66
  Bottom 0.406: C12.1 106.68,33.02 R35.P$2
N$67
  Bottom 0.406: C8.P$1 101.6,45.72 91.44,45.72 R27.P$2
N$68
  Bottom 0.406: 91.44,27.94 R27.P$1 | 91.44,27.94 R28.P$1 | 91.44,27.94 91.44,17.78 96.52,17.78 96.44,17.7 96.44,17.14 S5.4
N$69
  Bottom 0.406: C10.P$1 114.34,43.22 IC2.1
N$70
  Bottom 0.406: C15.1 114.3,12.7 IC3.1
N$71
  Bottom 0.406: 132.08,0.64 132.08,7.62 127,7.62 R38.P$2 121.92,12.7 IC3.8 121.88,10.2 C15.2 | R40.P$1 147.96,12.7 147.96,0.64 132.08,0.64 | 132.08,0.64 78.74,0.64 78.74,12.7 S4.S
N$72
  Bottom 0.406: S4.P 81.28,15.24 81.28,56.52 74.93,56.52 74.93,68.58 R39.P$1
N$73  (via drill 0.6)
  Top 0.406: v119.38,51.44 v114.3,51.44
  Bottom 0.406: R32.P$1 139.7,38.1 139.7,43.18 IC2.8 119.34,47.66 C10.P$2 119.34,50.76 v119.38,51.44 | R31.P$1 R30.P$2 | S4.O 83.82,58.42 76.2,58.42 76.2,63.5 R30.P$2 | v114.3,51.44 91.44,51.44 91.44,63.5 R30.P$2
N$74
  Bottom 0.406: C11.1 137.16,88.27 88.9,88.27 R31.P$2 R39.P$2
N$75  (via drill 0.6)
  Top 0.406: v53.34,40.64 v53.34,60.96 | v91.44,76.2 48.26,76.2 48.26,66.04 Q6.C
  Bottom 0.406: 111.76,78.74 111.76,73.66 114.3,73.66 114.3,68.58 IC5.6 | 147.96,43.18 147.96,68.58 | R44.P$2 147.96,43.18 | 147.96,43.18 147.96,27.94 R32.P$2 R40.P$2 144.78,17.78 S6.O | Q5.C 147.96,68.58 | 147.96,68.58 147.96,87.63 141.6,87.63 141.6,82.55 135.25,82.55 135.25,87.63 111.76,87.63 | 111.76,87.63 91.44,87.63 v91.44,76.2 | 111.76,78.74 SPEAKER_NEG1.1 111.76,87.63 | C17.1 111.76,78.74 | IC1.3 v53.34,40.64 | v53.34,60.96 53.34,66.04 Q6.C
N$76
  Bottom 0.406: C11.2 VR7-VOLUME.3
N$77
  Bottom 0.406: R1-22.P$2 R1-23.P$1
N$78
  Bottom 0.406: R42.P$2 127,73.66 | IC5.3 119.38,69.21 127,69.21 | 127,69.21 127,73.66 | 127,73.66 R41.P$1 ADDED1.P$2 | ADDED.P$1 132.08,69.21 127,69.21
N$79
  Bottom 0.406: AUDIO_R1.1 132.08,48.26 ADDED.P$2 132.08,56.52 134.62,56.52 134.62,86.36 124.46,86.36 R41.P$2
N$80
  Bottom 0.406: C18.P$1 124.46,63.5 IC5.1
N$81
  Bottom 0.406: IC5.7 102.23,66.04 102.23,83.82 | SPEAKER_POS1.1 102.23,83.82 | 102.23,83.82 C19.1
N$82
  Bottom 0.406: C19.2 104.14,71.12 R45.P$1 IC5.5
N$84
  Bottom 0.406: C20.1 106.68,55.88 R45.P$2
N$85  (via drill 0.6)
  Top 0.406: v116.2,66.04 116.2,86.36 73.66,86.36 73.66,81.28 ADDED_C.1
  Bottom 0.406: R43.P$2 129.54,67.94 121.92,67.94 121.92,66.04 IC5.2 v116.2,66.04
N$86
  Bottom 0.406: C16.1 R43.P$1
N$87
  Bottom 0.406: SP1.+ PIEZO_GND.1
N$88
  Bottom 0.406: SP1.- PIEZO_PLUS.1
N$89
  Bottom 0.406: S6.P 134.62,15.24 134.62,25.4 JACK_POS1.1
N$90
  Bottom 0.406: V1.+ V2.+ +9_BATT.1
N$91
  Bottom 0.406: Q5.B 142.24,71.12 142.24,65.41 144.78,65.41 | 144.78,65.41 147.32,65.41 147.32,53.34 R44.P$1 | 144.78,65.41 D4.P$1
N$92
  Bottom 0.406: SP2.- SPEAKER_POS.1
N$93
  Bottom 0.406: SP2.+ SPEAKR_NEG.1
N$94
  Bottom 0.406: JACK_POS.1 J1.+
N$95
  Bottom 0.406: +9_BATT1.1 233.04,83.82 J1.S
N$96
  Bottom 0.406: JACK_GND1.1 V1.- V2.- GND_BATT.1
N$97
  Bottom 0.406: J1.- JACK_GND.1
N$98
  Bottom 0.406: AUDIO_L.1 191.91,88.9 OUTPUT.SHIELD
N$99
  Bottom 0.406: OUTPUT.TIP AUDIO_R.1
N$100
  Bottom 0.406: OUTPUT.RING1 184.19,83.86 AUDIO_GND.1
N$101  (via drill 0.6)
  Top 0.406: v68.58,34.29 55.88,34.29 v55.88,60.96
  Bottom 0.406: S3.S 68.58,12.7 v68.58,34.29 | Q6.B 55.88,68.58 v55.88,60.96
N$102
  Bottom 0.406: ADDED_C1.1 53.34,72.39 | Q6.E 53.34,71.12 53.34,72.39 | 53.34,72.39 63.5,72.39 R46.P$1
N$103
  Bottom 0.406: R46.P$2 63.5,81.28 58.42,81.28 Q8.B
N$104
  Bottom 0.406: Q8.C 68.58,86.36 ADDED_C.2
N$105
  Bottom 0.406: R1-24.P$1 R1-23.P$2
N$106
  Bottom 0.406: R1-24.P$2 BOTTOM_NOTE.1
N$202
  Bottom 0.406: TOP_NOTE.1 PR1-INTONATION.S
(copper drawn outside any net)
  shapes: Bottom area x79, Bottom circle x4

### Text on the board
tPlace: 1 | 2 | 3 | 4 | 5 | 6 | 7 | 8 | 9 | 10 | 11 | 7 | 7 | 6 | 6 | 5 | 5 | 4 | 4 | 3 | 3 | 2 | 2 | 1 | 1 | 1 | 2 | 3 | 4 | 5 | 6 | 7 | 8 | 9 | 10 | 11
tNames: SENS | 2X FILTER | POWER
